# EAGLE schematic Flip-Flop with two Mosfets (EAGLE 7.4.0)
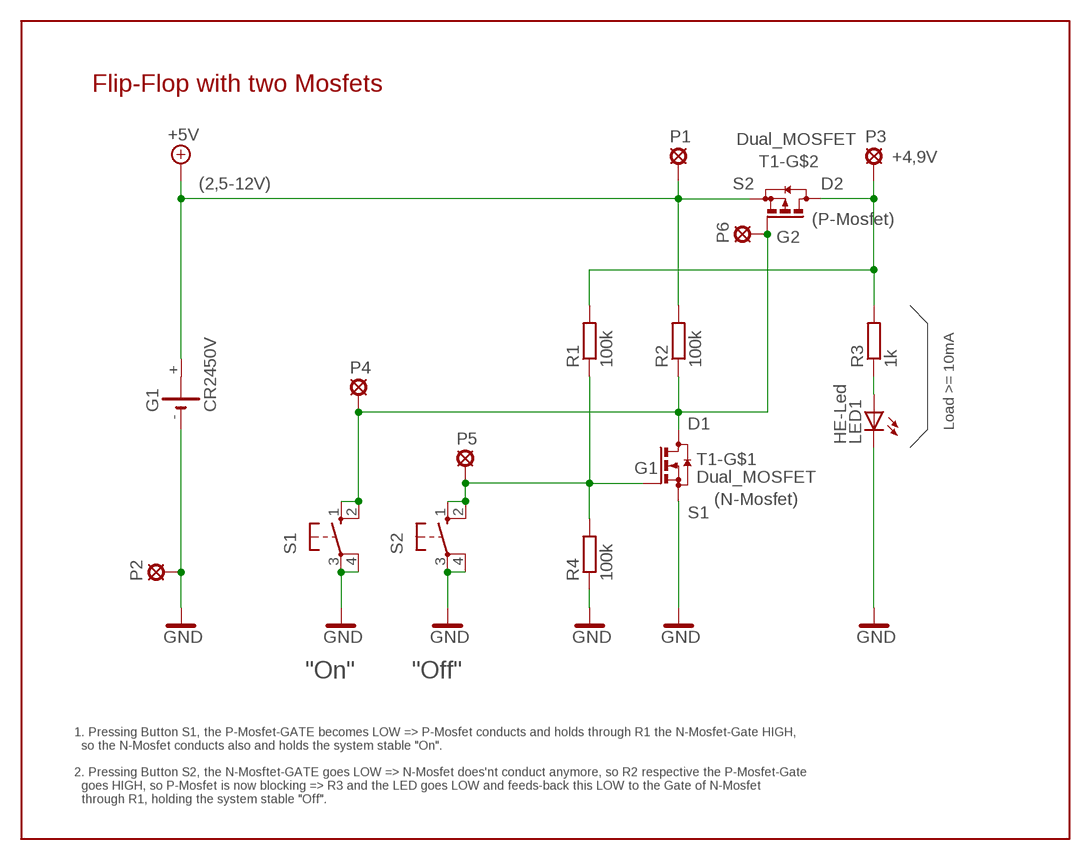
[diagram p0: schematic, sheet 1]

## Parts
G1  CR2450V  [CR2450V]
LED1  HE-Led  LED3MM  [LED3MM]
P1  5V  LSP10  [LSP10]
P2  GND  LSP10  [LSP10]
P3  4,5V-Out  LSP10  [LSP10]
P4  On  LSP10  [LSP10]
P5  Off  LSP10  [LSP10]
P6  D1G2  LSP10  [LSP10]
R1  100k  R-EU_R0805  [R0805]
R2  100k  R-EU_R0805  [R0805]
R3  1k  R-EU_R0805  [R0805]
R4  100k  R-EU_R0805  [R0805]
S1  10-XX  [B3F-10XX]
S2  10-XX  [B3F-10XX]
T1-  Dual_MOSFET  NP_MOSFET_SOT23-6  [SOT23-6]

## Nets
+5V: G1.+ P1.MP R2.2 T1-.2(S)
GND: G1.- LED1.K(C) P2.MP R4.1 S1.3(P) S1.4(P1) S2.3(P) S2.4(P1) T1-.5(S)
N$1: P5.MP R1.1 R4.2 S2.1(S) S2.2(S1) T1-.1(G)
N$2: LED1.A R3.1
N$3: P4.MP P6.MP R2.1 S1.1(S) S1.2(S1) T1-.3(G) T1-.6(D)
N$4: P3.MP R1.2 R3.2 T1-.4(D)
Unconnected: G1.+@1(+)

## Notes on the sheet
- Flip-Flop with two Mosfets
- +4,9V
- (2,5-12V) | S2 | D2
- (P-Mosfet)
- G2
- D1 | Load >= 10mA
- G1
- (N-Mosfet)
- S1
- "On" | "Off"
- 1. Pressing Button S1, the P-Mosfet-GATE becomes LOW => P-Mosfet conducts and holds through R1 the N-Mosfet-Gate HIGH,
    so the N-Mosfet conducts also and holds the system stable "On".
- 2. Pressing Button S2, the N-Mosftet-GATE goes LOW => N-Mosfet does'nt conduct anymore, so R2 respective the P-Mosfet-Gate
    goes HIGH, so P-Mosfet is now blocking => R3 and the LED goes LOW and feeds-back this LOW to the Gate of N-Mosfet
    through R1, holding the system stable "Off".

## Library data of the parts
G1 = battery:CR2450V: LI BATTERY Varta
LED1 = led:LED: LED
P1-P6 = solpad:LSP10: SOLDER PAD
R1-R4 = rcl1:R-EU_: RESISTOR, European symbol
S1 S2 = switch-omron:10-XX: OMRON SWITCH; MPN: B3F-1000; OC_FARNELL: 176432; OC_NEWARK: 36M3542
T1- = transistor-small-signal:NP_MOSFET_SOT23-6: Dual N- & P-Channel Mosfet 20V / ~2A / ~1W / ~100mO / SOT23-6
